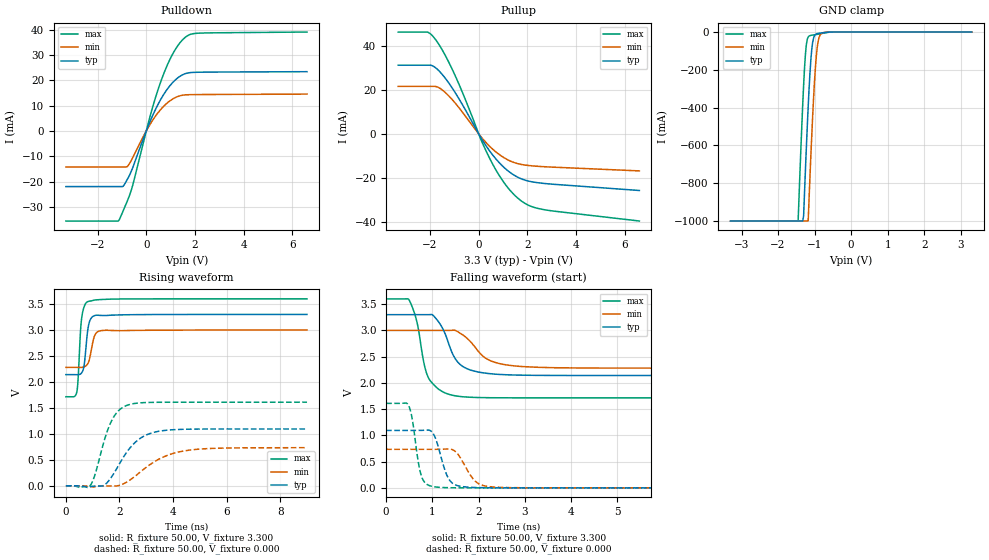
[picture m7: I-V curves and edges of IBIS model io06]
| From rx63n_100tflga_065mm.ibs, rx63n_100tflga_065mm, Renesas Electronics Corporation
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[Model]   io06
Model_type   I/O
Polarity   Non-Inverting
Enable   Active-High
Vinl  =   0.660V
Vinh  =   2.640V
Vmeas =   1.650V
Cref  =   30.00pF
| variable   typ   min   max
C_comp   3.380pF   3.380pF   3.380pF
| variable   typ   min   max
[Temperature Range]   45.000   105.000   -40.000
| variable   typ   min   max
[Voltage Range]   3.300V   3.000V   3.600V
| variable   typ   min   max
[Pullup Reference]   3.300V   3.000V   3.600V
| variable   typ   min   max
[Pulldown Reference]   0.000V   0.000V   0.000V
| variable   typ   min   max
[POWER Clamp Reference] 3.300V   3.000V   3.600V
| variable   typ   min   max
[GND Clamp Reference]   0.000V   0.000V   0.000V
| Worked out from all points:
|   slope of the pulldown table from 0 to 0.495 V, typ, clamps not added: 46.2 ohm
|   slope of the pullup table from 0 to 0.495 V, typ, clamps not added: 58.5 ohm
|   GND clamp passes 1 mA (typ) near -0.63 V on its own axis
|   rising waveform, R_fixture 50.00, V_fixture 3.300: 20-80 % time 144ps typ, 176ps min, 128ps max; typ from 2.14 V to 3.3 V
|   rising waveform, R_fixture 50.00, V_fixture 0.000: 20-80 % time 909ps typ, 1.31ns min, 596ps max; typ from 0 V to 1.09 V
|   falling waveform, R_fixture 50.00, V_fixture 3.300: 20-80 % time 372ps typ, 511ps min, 270ps max; typ from 3.3 V to 2.14 V
|   falling waveform, R_fixture 50.00, V_fixture 0.000: 20-80 % time 230ps typ, 311ps min, 164ps max; typ from 1.09 V to 0 V
[Pulldown]
| io06 Pulldown rx631_rx63n
| Thu Mar 22 17:15:49 2012
| voltage   I(typ)   I(min)   I(max)
-3.3V     -21.93mA   -14.19mA   -35.51mA
-1.125V   -21.93mA   -14.19mA   -35.28mA
-950mV    -21.8mA    -14.19mA   -31.51mA
-725mV    -18.13mA   -13.36mA   -26.35mA
-525mV    -13.67mA   -9.89mA    -20.27mA
200mV     4.744mA    3.297mA    7.31mA
600mV     12.56mA    8.559mA    19.59mA
1.1V      19.27mA    12.7mA     30.64mA
1.375V    21.53mA    13.87mA    34.7mA
1.6V      22.62mA    14.25mA    36.95mA
2.2V      23.2mA     14.39mA    38.62mA
6.6V      23.41mA    14.56mA    39.05mA
[Pullup]
| io06 Pullup rx631_rx63n
| Thu Mar 22 17:15:49 2012
| voltage   I(typ)   I(min)   I(max)
-3.3V     31.12mA    21.48mA    46.18mA
-2.1V     31.12mA    21.48mA    46.13mA
-1.75V    29.8mA     21.42mA    42.5mA
-1.425V   26mA       19.27mA    36.71mA
-950mV    18.45mA    13.76mA    26.08mA
100mV     -1.895mA   -1.397mA   -2.764mA
575mV     -9.625mA   -6.998mA   -13.77mA
1.125V    -16.13mA   -11.44mA   -23.43mA
1.7V      -20.25mA   -13.86mA   -30.1mA
2.1V      -21.66mA   -14.51mA   -32.76mA
2.7V      -22.61mA   -15mA      -34.53mA
6.6V      -25.8mA    -16.9mA    -39.66mA
[GND Clamp]
| io06 GNDClamp rx631_rx63n
| Thu Mar 22 17:15:49 2012
| voltage   I(typ)   I(min)   I(max)
-3.3V     -1A        -1A        -1A
-1.45V    -1A        -1A        -998.8mA
-1.325V   -1A        -1A        -385.7mA
-1.3V     -971.8mA   -1A        -281.5mA
-1.25V    -727.5mA   -1A        -116.3mA
-1.175V   -394.3mA   -998.4mA   -26.13mA
-1.15V    -297.8mA   -877.6mA   -21.18mA
-1.075V   -87.77mA   -537.8mA   -16.82mA
-975mV    -12.8mA    -181.3mA   -13.72mA
-900mV    -7.379mA   -46.43mA   -11.41mA
-825mV    -5.325mA   -9.739mA   -8.6mA
3.3V      0A         0A         0A
[POWER Clamp]
| io06 PWRClamp rx631_rx63n
| Thu Mar 22 17:15:49 2012
| voltage   I(typ)   I(min)   I(max)
-3.3V     0A         0A         0A
0V        0A         0A         0A
3.3V      0A         0A         0A
[Ramp]
dV/dt_r   0.657/908.19p  0.440/1.31n   0.966/594.87p
dV/dt_f   0.696/371.64p  0.432/508.54p  1.131/269.92p
R_load = 50.00ohm
[Rising Waveform]
| io06 Rising-High rx631_rx63n
| Thu Mar 22 17:15:49 2012
R_fixture = 50.00
V_fixture = 3.300
V_fixture_min = 3.000
V_fixture_max = 3.600
C_fixture = 0.00pF
| Time   V(typ)   V(min)   V(max)
0s        2.141V     2.28V      1.715V
405ps     2.14V      2.28V      1.8V
450ps     2.139V     2.28V      2.011V
580ps     2.17V      2.28V      3.19V
685ps     2.336V     2.291V     3.453V
800ps     2.932V     2.338V     3.543V
900ps     3.186V     2.483V     3.558V
1.08ns    3.278V     2.899V     3.577V
1.315ns   3.281V     2.988V     3.587V
9ns       3.3V       3V         3.6V
[Rising Waveform]
| io06 Rising-Low rx631_rx63n
| Thu Mar 22 17:15:49 2012
R_fixture = 50.00
V_fixture = 0.000
C_fixture = 0.00pF
| Time   V(typ)   V(min)   V(max)
0s        0V         0V         0V
915ps     -16mV      -15mV      10mV
1.09ns    -7mV       -20mV      220mV
1.4ns     4mV        -4mV       813mV
1.675ns   147mV      -4mV       1.218V
1.94ns    370mV      1mV        1.433V
2.305ns   671mV      82mV       1.554V
3.045ns   988mV      373mV      1.604V
4.39ns    1.088V     669mV      1.609V
9ns       1.094V     734mV      1.61V
[Falling Waveform]
| io06 Falling-High rx631_rx63n
| Thu Mar 22 17:15:49 2012
R_fixture = 50.00
V_fixture = 3.300
V_fixture_min = 3.000
V_fixture_max = 3.600
C_fixture = 0.00pF
| Time   V(typ)   V(min)   V(max)
0s        3.3V       3V         3.6V
490ps     3.3V       3V         3.589V
665ps     3.3V       3V         3.163V
900ps     3.3V       3V         2.125V
1.17ns    3.118V     3V         1.859V
1.385ns   2.667V     3V         1.775V
1.755ns   2.268V     2.846V     1.73V
2.17ns    2.183V     2.462V     1.718V
2.74ns    2.151V     2.327V     1.715V
9ns       2.141V     2.28V      1.715V
[Falling Waveform]
| io06 Falling-Low rx631_rx63n
| Thu Mar 22 17:15:49 2012
R_fixture = 50.00
V_fixture = 0.000
C_fixture = 0.00pF
| Time   V(typ)   V(min)   V(max)
0s        1.094V     734mV      1.61V
480ps     1.094V     734mV      1.577V
560ps     1.094V     734mV      1.332V
755ps     1.095V     734mV      249mV
1.005ns   1.05V      734mV      26mV
1.34ns    194mV      740mV      3mV
1.645ns   24mV       513mV      1mV
1.95ns    6mV        110mV      0V
2.33ns    1mV        15mV       0V
9ns       0V         0V         0V
